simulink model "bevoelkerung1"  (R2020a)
settings: Solver=ode45  StartTime=0.0  StopTime=200  MaxStep=4  RelTol=1e-3  EnableMultiTasking=on

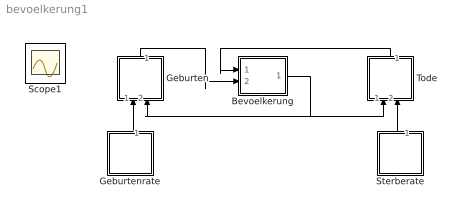
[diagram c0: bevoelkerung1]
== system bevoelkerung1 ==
  Bevoelkerung : Subsystem  mask{m0=10}
      mask prompts: m0 "Anfangswert"
  Geburten : Subsystem
  Geburtenrate : Subsystem  mask{k=0.03}
      mask prompts: k "Constant"
  Sterberate : Subsystem  mask{k=0.01}
      mask prompts: k "Constant"
  Tode : Subsystem
  Scope1 : Scope
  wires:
  Geburtenrate/1(Out1) -> Geburten/1(In1)
  Geburten/1(Out1) -> Bevoelkerung/2(In2)
  Bevoelkerung/1(Out1) -> Geburten/2(In2), Tode/1(In1)
  Sterberate/1(Out1) -> Tode/2(In2)
  Tode/1(Out1) -> Bevoelkerung/1(In1)

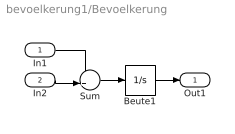
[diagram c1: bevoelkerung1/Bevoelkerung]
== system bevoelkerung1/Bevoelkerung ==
  In1 : Inport
  In2 : Inport  Port=2
  Beute1 : Integrator  InitialCondition=m0
  Sum : Sum  Inputs=-+|  SaturateOnIntegerOverflow=on
  Out1 : Outport
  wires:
  Sum/1 -> Beute1/1
  In1/1 -> Sum/1
  Beute1/1 -> Out1/1
  In2/1 -> Sum/2

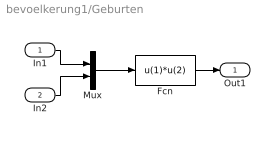
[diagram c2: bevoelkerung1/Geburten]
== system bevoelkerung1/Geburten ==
  In1 : Inport
  In2 : Inport  Port=2
  Fcn : Fcn  Expr=u(1)*u(2)
  Mux : Mux  Inputs=2
  Out1 : Outport
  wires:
  Fcn/1 -> Out1/1
  Mux/1 -> Fcn/1
  In1/1 -> Mux/1
  In2/1 -> Mux/2

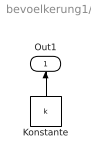
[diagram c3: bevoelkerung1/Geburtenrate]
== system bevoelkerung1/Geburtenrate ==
  Konstante : Constant  Value=k
  Out1 : Outport
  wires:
  Konstante/1 -> Out1/1

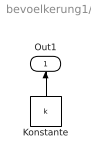
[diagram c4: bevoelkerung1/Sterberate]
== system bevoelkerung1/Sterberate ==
  Konstante : Constant  Value=k
  Out1 : Outport
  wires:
  Konstante/1 -> Out1/1

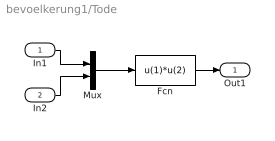
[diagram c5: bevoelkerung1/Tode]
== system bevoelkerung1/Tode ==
  In1 : Inport
  In2 : Inport  Port=2
  Fcn : Fcn  Expr=u(1)*u(2)
  Mux : Mux  Inputs=2
  Out1 : Outport
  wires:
  Fcn/1 -> Out1/1
  Mux/1 -> Fcn/1
  In1/1 -> Mux/1
  In2/1 -> Mux/2
